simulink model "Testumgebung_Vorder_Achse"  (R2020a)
settings: Solver=ode4  StartTime=0.0  StopTime=30.0  FixedStep=0.01  RelTol=1e-3
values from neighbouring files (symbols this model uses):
  Achsschraeglaufwinkel_v_value = 1    [Single_Testskript_Vorderachse.m]    (also in Testskript_Vorderachse.m = (b-a).*rand(1,1) + a)
  cv = 80000    [Single_Testskript_Vorderachse.m]    (also in Testskript_Vorderachse.m = (b-a).*rand(1,1) + a)
  Fahrerlenkwinkel_v_value = 0.3    [Single_Testskript_Vorderachse.m]    (also in Testskript_Vorderachse.m = (b-a).*rand(1,1) + a)
  Geschwindigkeit_value = 8.33    [Single_Testskript_Vorderachse.m]    (also in Testskript_Vorderachse.m = (b-a).*rand(1,1) + a)
  Gierrate_value = 2    [Single_Testskript_Vorderachse.m]    (also in Testskript_Vorderachse.m = (b-a).*rand(1,1) + a; Single_TestSkript_Hinterachse.m; Testskript_Hinterachse.m = (b-a).*rand(1,1) + a; Single_Testskript_Karosserie.m)
  lv = 1.5    [Single_Testskript_Vorderachse.m]    (also in Testskript_Vorderachse.m = (b-a).*rand(1,1) + a; Single_Testskript_Karosserie.m = 1.3; Testskript_Karosserie.m = (b-a).*rand(1,1) + a)
  Schwimmwinkel_value = 1.3    [Single_Testskript_Vorderachse.m]    (also in Testskript_Vorderachse.m = (b-a).*rand(1,1) + a; Single_TestSkript_Hinterachse.m; Testskript_Hinterachse.m = (b-a).*rand(1,1) + a; Testskript_Ausgabe.m = (b-a).*rand(1,1) + a)

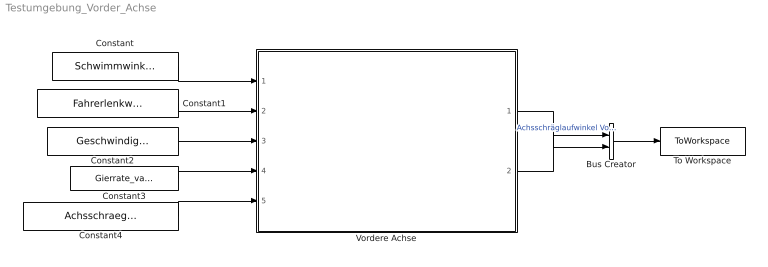
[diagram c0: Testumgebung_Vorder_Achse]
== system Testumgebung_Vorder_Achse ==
  Bus Creator : BusCreator  Inputs=2
  Constant : Constant  Value=Schwimmwinkel_value
  Constant1 : Constant  Value=Fahrerlenkwinkel_v_value
  Constant2 : Constant  Value=Geschwindigkeit_value
  Constant3 : Constant  Value=Gierrate_value
  Constant4 : Constant  Value=Achsschraeglaufwinkel_v_value
  To Workspace : ToWorkspace  VariableName=simout  SaveFormat=Timeseries  SampleTime=-1
  Vordere Achse : Subsystem
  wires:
  Constant/1 -> Vordere Achse/1(Schwimmwinkel beta)
  Constant1/1 -> Vordere Achse/2(Fahrerlenkwinkel teta_v)
  Constant2/1 -> Vordere Achse/3(Geschwindigkeit KvCx)
  Constant4/1 -> Vordere Achse/5(Achsschräglaufwinkel vornerachse Alpha_v)
  Constant3/1 -> Vordere Achse/4(Gierrate K_psi_punkt)
  Vordere Achse/1(Achsschräglaufwinkel vorderachse Alpha_v) -> Bus Creator/1  "Achsschräglaufwinkel Vorderachse Alpha_v"
  Vordere Achse/2(Seitenführungskraft vorderachse RFyv) -> Bus Creator/2
  Bus Creator/1 -> To Workspace/1

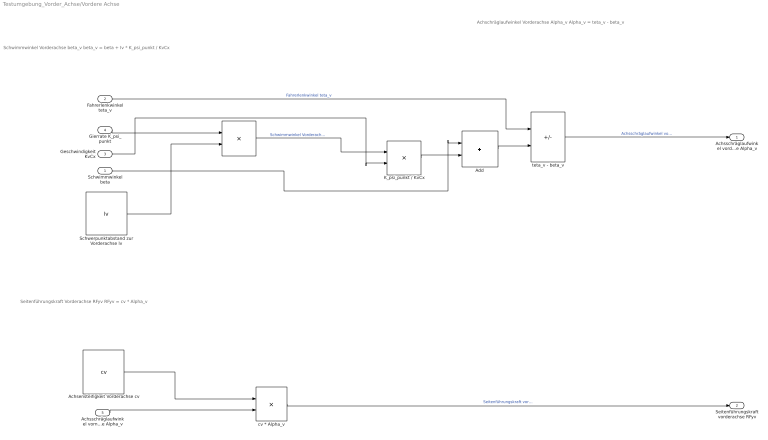
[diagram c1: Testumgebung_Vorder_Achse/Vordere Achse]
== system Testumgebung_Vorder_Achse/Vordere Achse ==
  note: Seitenführungskraft Vorderachse RFyv RFyv = cv * Alpha_v
  note: Schwimmwinkel Vorderachse beta_v beta_v = beta + Iv * K_psi_punkt / KvCx
  note: Achschräglaufwinkel Vorderachse Alpha_v Alpha_v = teta_v - beta_v
  Schwimmwinkel beta : Inport
  Fahrerlenkwinkel teta_v : Inport  Port=2
  Geschwindigkeit KvCx : Inport  Port=3
  Gierrate K_psi_punkt : Inport  Port=4
  Achsschräglaufwinkel vornerachse Alpha_v : Inport  Port=5
  " " : Product  Inputs=**
  Achsensteifigkeit Vorderachse cv : Constant  Value=cv
  Add : Sum
  K_psi_punkt / KvCx : Product  Inputs=*/
  Schwerpunktabstand zur Vorderachse lv : Constant  Value=lv
  cv * Alpha_v : Product
  teta_v - beta_v : Sum  Inputs=+-
  Achsschräglaufwinkel vorderachse Alpha_v : Outport
  Seitenführungskraft vorderachse RFyv : Outport  Port=2
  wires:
  teta_v - beta_v/1 -> Achsschräglaufwinkel vorderachse Alpha_v/1  "Achsschräglaufwinkel vorderachse Alpha_v"
  cv * Alpha_v/1 -> Seitenführungskraft vorderachse RFyv/1  "Seitenführungskraft vorderachse RFyv"
  Achsensteifigkeit Vorderachse cv/1 -> cv * Alpha_v/1
  Achsschräglaufwinkel vornerachse Alpha_v/1 -> cv * Alpha_v/2
  " "/1 -> K_psi_punkt / KvCx/1  "Schwimmwinkel Vorderachse beta_v"
  Geschwindigkeit KvCx/1 -> K_psi_punkt / KvCx/2
  Fahrerlenkwinkel teta_v/1 -> teta_v - beta_v/1  "Fahrerlenkwinkel teta_v"
  Schwimmwinkel beta/1 -> Add/1
  K_psi_punkt / KvCx/1 -> Add/2
  Add/1 -> teta_v - beta_v/2
  Gierrate K_psi_punkt/1 -> " "/1
  Schwerpunktabstand zur Vorderachse lv/1 -> " "/2
